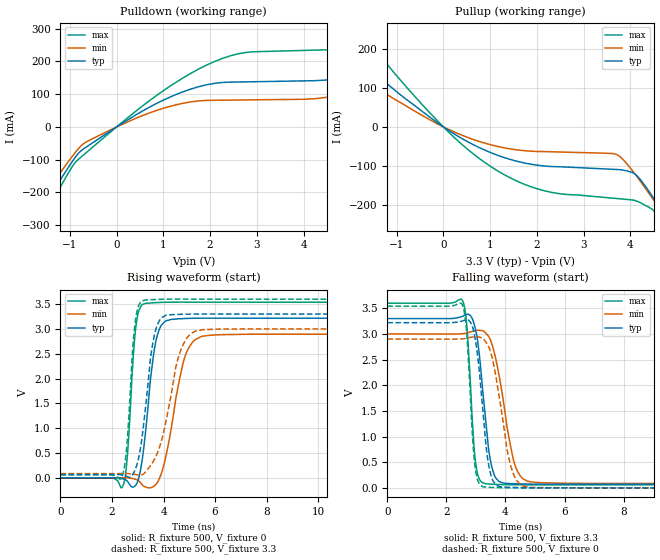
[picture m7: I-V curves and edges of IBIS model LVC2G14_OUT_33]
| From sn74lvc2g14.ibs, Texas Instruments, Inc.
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[Model]   LVC2G14_OUT_33
Model_type  Output
Vref =   0
Rref =   500
Cref =   50p
Vmeas =   1.5
| variable   typ   min   max
C_comp   9.43pF   5.86pF   12.62pF
| C_pullup   9.92pF   5.86pF   11.98pF
| C_pulldown   8.95pF   6.08pF   12.62pF
[Temperature Range]   40   100   -40
| Ambient temperature   25   85   -40
[Voltage range]   3.3   3   3.6
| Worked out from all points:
|   slope of the pulldown table from 0 to 0.495 V, typ, clamps not added: 11.3 ohm
|   slope of the pullup table from 0 to 0.495 V, typ, clamps not added: 13.6 ohm
|   rising waveform, R_fixture 500, V_fixture 0: 20-80 % time 398ps typ, 609ps min, 249ps max; typ from 0 V to 3.22 V
|   falling waveform, R_fixture 500, V_fixture 3.3: 20-80 % time 336ps typ, 516ps min, 215ps max; typ from 3.3 V to 0.069 V
|   rising waveform, R_fixture 500, V_fixture 3.3: 20-80 % time 424ps typ, 697ps min, 257ps max; typ from 0.069 V to 3.3 V
|   falling waveform, R_fixture 500, V_fixture 0: 20-80 % time 321ps typ, 486ps min, 210ps max; typ from 3.22 V to 0 V
[Pulldown]
| LVC2G14_OUT_33
|   Voltage   I(typ)   I(min)   I(max)
-5.5V     -1.112A    -993.8mA   -1.259A
-2.645V   -490.3mA   -433.2mA   -553.8mA
-1.49V    -226.9mA   -197.7mA   -257.3mA
-540mV    -51.04mA   -37.69mA   -65.27mA
1.025V    83.38mA    58mA       112.9mA
2.285V    136mA      81.66mA    210.1mA
4.75V     148.7mA    96.8mA     237.9mA
6.98V     278.7mA    201.6mA    396.3mA
7.35V     308.5mA    129.4mA    437mA
7.84V     330.1mA    92.52mA    494.2mA
8.75V     170.8mA    93.27mA    500.6mA
11V       160mA      96.49mA    276.8mA
[Pullup]
| LVC2G14_OUT_33
|   Voltage   I(typ)   I(min)   I(max)
-5.5V     609.5mA    479.2mA    854.2mA
-3.13V    322.5mA    249.3mA    458mA
-2.385V   237.2mA    181.8mA    339.2mA
-1.845V   177.9mA    135.2mA    255.8mA
-130mV    10.97mA    8.025mA    16.16mA
1.04V     -67.46mA   -46.7mA    -103.9mA
2.145V    -100.4mA   -63.42mA   -163.8mA
3.71V     -109.5mA   -71.26mA   -184.2mA
4.15V     -126.7mA   -129.5mA   -191.6mA
4.765V    -233mA     -235.6mA   -263.4mA
4.95V     -268.4mA   -268.9mA   -301.3mA
11V       -1.523A    -1.428A    -1.684A
[Ramp]
| LVC2G14_OUT_33
| variable   typ   min   max
dV/dt_r   2.04/4.30E-10   1.86/6.66E-10   2.24/2.69E-10
dV/dt_f   1.99/3.62E-10   1.79/5.54E-10   2.17/2.30E-10
R_load = 500
[Rising Waveform]
| LVC2G14_OUT_33
R_fixture =   500
C_fixture =   0
L_fixture =   0
V_fixture =   0
V_fixture_min = 0
V_fixture_max = 0
|   Time   V(typ)   V(min)   V(max)
0s        141.8pV    4.978nV    2.659nV
2.425ns   -17.72mV   1.578mV    -161.8mV
2.595ns   -65.3mV    1.024mV    431.9mV
2.925ns   -145.1mV   -30.22mV   3.038V
3.295ns   886.7mV    -182.1mV   3.516V
3.625ns   2.523V     -167.4mV   3.528V
3.875ns   3.037V     29.95mV    3.535V
4.79ns    3.21V      2.371V     3.54V
5.5ns     3.218V     2.853V     3.539V
24.99ns   3.216V     2.894V     3.539V
[Falling Waveform]
| LVC2G14_OUT_33
R_fixture =   500
C_fixture =   0
L_fixture =   0
V_fixture =   3.3
V_fixture_min = 3
V_fixture_max = 3.6
|   Time   V(typ)   V(min)   V(max)
0s        3.3V       3V         3.6V
2.545ns   3.345V     3.004V     3.651V
2.695ns   3.381V     3.021V     3.127V
2.985ns   3.089V     3.065V     506.7mV
3.32ns    1.378V     3.025V     81.85mV
3.47ns    601.1mV    2.912V     72.43mV
3.67ns    194.1mV    2.518V     67.01mV
4.27ns    81.2mV     547.2mV    59.72mV
4.79ns    72.94mV    123.6mV    58.51mV
24.99ns   69.39mV    85.93mV    58.96mV
[Rising Waveform]
| LVC2G14_OUT_33
R_fixture =   500
C_fixture =   0
L_fixture =   0
V_fixture =   3.3
V_fixture_min = 3
V_fixture_max = 3.6
|   Time   V(typ)   V(min)   V(max)
0s        69.35mV    85.87mV    58.92mV
2.375ns   61.47mV    87.01mV    2.779mV
2.57ns    32.95mV    87.13mV    611.2mV
2.89ns    154.2mV    68.53mV    3.088V
3.18ns    865.1mV    64.73mV    3.57V
3.5ns     2.43V      251.6mV    3.589V
3.77ns    3.094V     513.6mV    3.596V
4.615ns   3.294V     2.491V     3.601V
5.27ns    3.3V       2.961V     3.6V
24.99ns   3.3V       3V         3.6V
[Falling Waveform]
| LVC2G14_OUT_33
R_fixture =   500
C_fixture =   0
L_fixture =   0
V_fixture =   0
V_fixture_min = 0
V_fixture_max = 0
|   Time   V(typ)   V(min)   V(max)
0s        3.22V      2.9V       3.542V
2.535ns   3.251V     2.903V     3.574V
2.685ns   3.276V     2.917V     3.038V
2.96ns    2.951V     2.945V     463.8mV
3.25ns    1.406V     2.903V     18.91mV
3.4ns     556.8mV    2.782V     10.32mV
3.58ns    134.6mV    2.457V     7.533mV
4.14ns    9.989mV    517.9mV    1.354mV
4.625ns   3.539mV    28.14mV    -211.6uV
24.99ns   39.55uV    47.02uV    34.51uV
